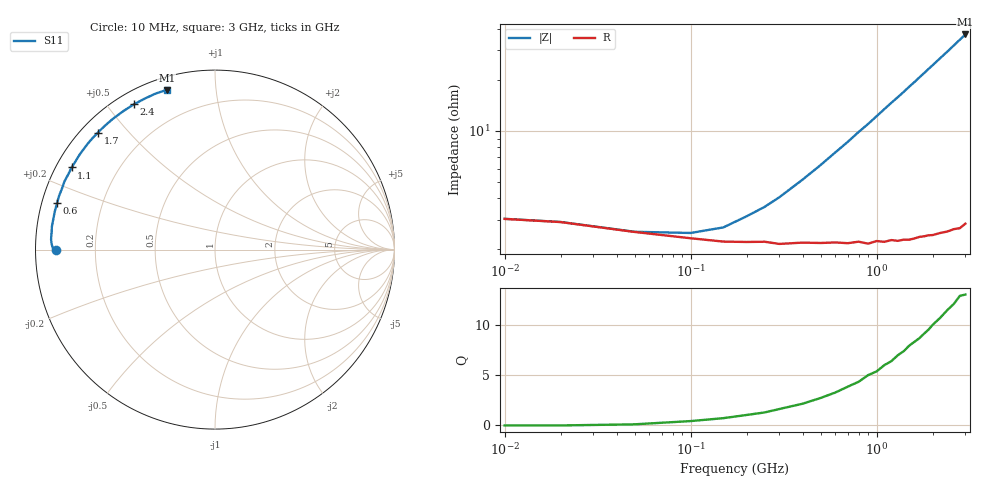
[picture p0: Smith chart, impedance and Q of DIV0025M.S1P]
! SIEMENS Small Signal Semiconductors
! BAV99
! Silicon Switching Diode in SOT23
! IF = 25 mA
! S-Parameters:  May  1995
# GHz  S  MA  R  50
!  f  S11
! GHz  MAG  ANG
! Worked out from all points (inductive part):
!   30 points, 10 MHz to 3 GHz, reference 50 ohm
!   read as one part to ground: L = 1.91 nH near 600 MHz
!   highest Q = 13.1 at 3 GHz (marker M1), where L = 1.97 nH
!   S11 on the Smith chart (normalised r, x): 10 MHz: 0.06, -0.00; 600 MHz: 0.04, +0.14; 1.1 GHz: 0.04, +0.27; 1.7 GHz: 0.05, +0.41; 2.4 GHz: 0.05, +0.59; 3 GHz: 0.06, +0.74
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0.01  0.8859 -179.7
0.02  0.8904 -179.7
0.05  0.9036 179.6
0.1  0.9112 177.9
0.15  0.915 176.5
0.2  0.9155 174.9
0.25  0.9153 173.6
0.3  0.9179 172.1
0.4  0.9167 169.3
0.5  0.9176 166.5
0.6  0.9175 163.7
0.7  0.9188 161.0
0.8  0.9179 158.2
0.9  0.9208 155.6
1  0.9188 152.9
1.1  0.9206 150.2
1.2  0.9197 147.6
1.3  0.9215 145.1
1.5  0.9225 140.0
1.6  0.9225 137.6
1.7  0.9222 135.1
1.9  0.9234 130.3
2  0.9245 128.0
2.2  0.9254 123.4
2.4  0.927 119.1
2.6  0.928 114.8
2.8  0.9303 110.7
3  0.9294 106.8
